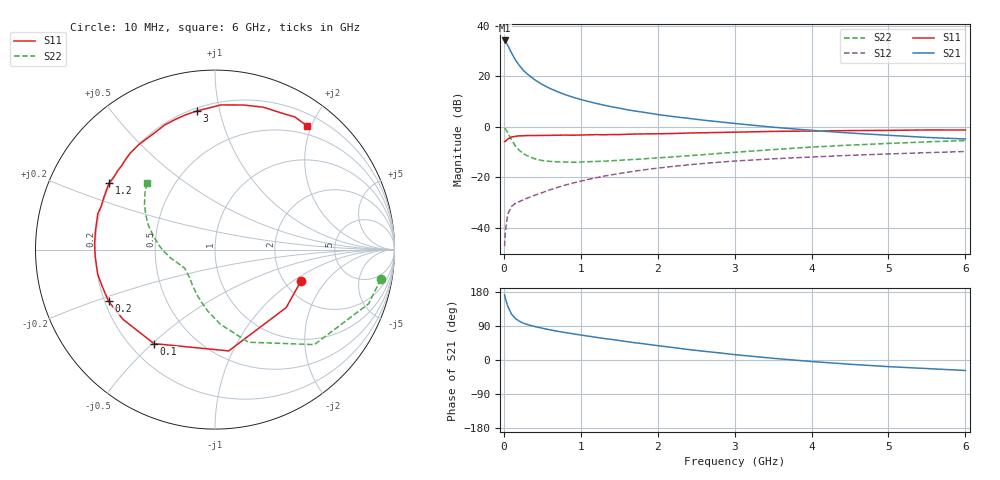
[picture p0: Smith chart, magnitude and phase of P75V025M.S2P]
! SIEMENS Small Signal Semiconductors
! BFP196
! Si NPN RF Bipolar Junction Transistor in SOT143
! VCE = 5 V  IC = 25 mA
! Common Emitter S-Parameters:  May  1996
# GHz  S  MA  R  50
!  f  S11  S21  S12  S22
! GHz  MAG  ANG  MAG  ANG  MAG  ANG  MAG  ANG
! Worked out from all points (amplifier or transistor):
!   36 points, 10 MHz to 6 GHz, reference 50 ohm
!   highest |S21| = 34.2 dB at 10 MHz (marker M1)
!   |S21| within 3 dB of that: start of sweep to 68.33 MHz
!   unconditionally stable (mu >= 1): 624.6 MHz to 3.456 GHz
!   at 250 MHz: K = 0.65, MSG = 25.7 dB, |S12| = -29.0 dB
!   at 1.4 GHz: K = 1.11, MAG = 11.5 dB, |S12| = -19.1 dB
!   at 6 GHz: K = 0.97, MSG = 2.5 dB, |S12| = -9.8 dB
!   S11 on the Smith chart (normalised r, x): 10 MHz: 2.44, -1.16; 100 MHz: 0.29, -0.51; 200 MHz: 0.22, -0.22; 1.2 GHz: 0.19, +0.28; 3 GHz: 0.22, +0.85; 6 GHz: 0.37, +1.94
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0.01  0.5097 -20.3  51.08 171.6  0.0043 85.4  0.938 -10.1
0.02  0.5116 -39.1  48.8 162.4  0.0085 77.5  0.9077 -19.4
0.05  0.5696 -82.3  41.24 142.0  0.0183 59.4  0.7659 -43.7
0.1  0.6244 -123.0  28.81 121.0  0.0263 47.1  0.5485 -70.2
0.15  0.6431 -142.7  21.04 109.6  0.0303 42.8  0.4163 -86.0
0.2  0.6593 -154.1  16.45 102.5  0.0328 42.8  0.3425 -97.1
0.25  0.6611 -162.3  13.28 97.5  0.0355 43.3  0.2948 -106.0
0.3  0.6677 -168.0  11.22 93.9  0.0382 45.6  0.267 -112.8
0.4  0.6687 -176.7  8.532 88.5  0.0438 48.4  0.2316 -123.3
0.5  0.6717 177.5  6.839 83.9  0.0495 50.5  0.2136 -130.8
0.6  0.6738 171.7  5.72 79.6  0.0562 52.9  0.2055 -136.4
0.7  0.6772 166.9  4.926 75.7  0.0629 54.1  0.2013 -140.7
0.8  0.6829 162.9  4.304 72.4  0.0699 54.6  0.1997 -144.3
1.1  0.6895 151.3  3.152 62.9  0.0906 54.7  0.2026 -151.3
1.2  0.6969 147.7  2.897 59.8  0.0974 54.3  0.2049 -153.4
1.6  0.7073 134.8  2.173 48.5  0.1246 51.2  0.2209 -160.1
2.2  0.7323 117.4  1.588 32.9  0.1636 44.3  0.2523 -169.4
3  0.7785 97.5  1.16 14.2  0.2087 34.0  0.311 176.1
3.5  0.8069 87.6  0.977 4.5  0.2311 27.6  0.3518 167.5
4.5  0.8379 71.2  0.749 -11.2  0.271 16.2  0.4319 153.3
5.5  0.8626 58.9  0.613 -22.6  0.306 5.5  0.5008 141.2
6  0.859 53.3  0.571 -27.7  0.3227 -0.3  0.5317 135.4
